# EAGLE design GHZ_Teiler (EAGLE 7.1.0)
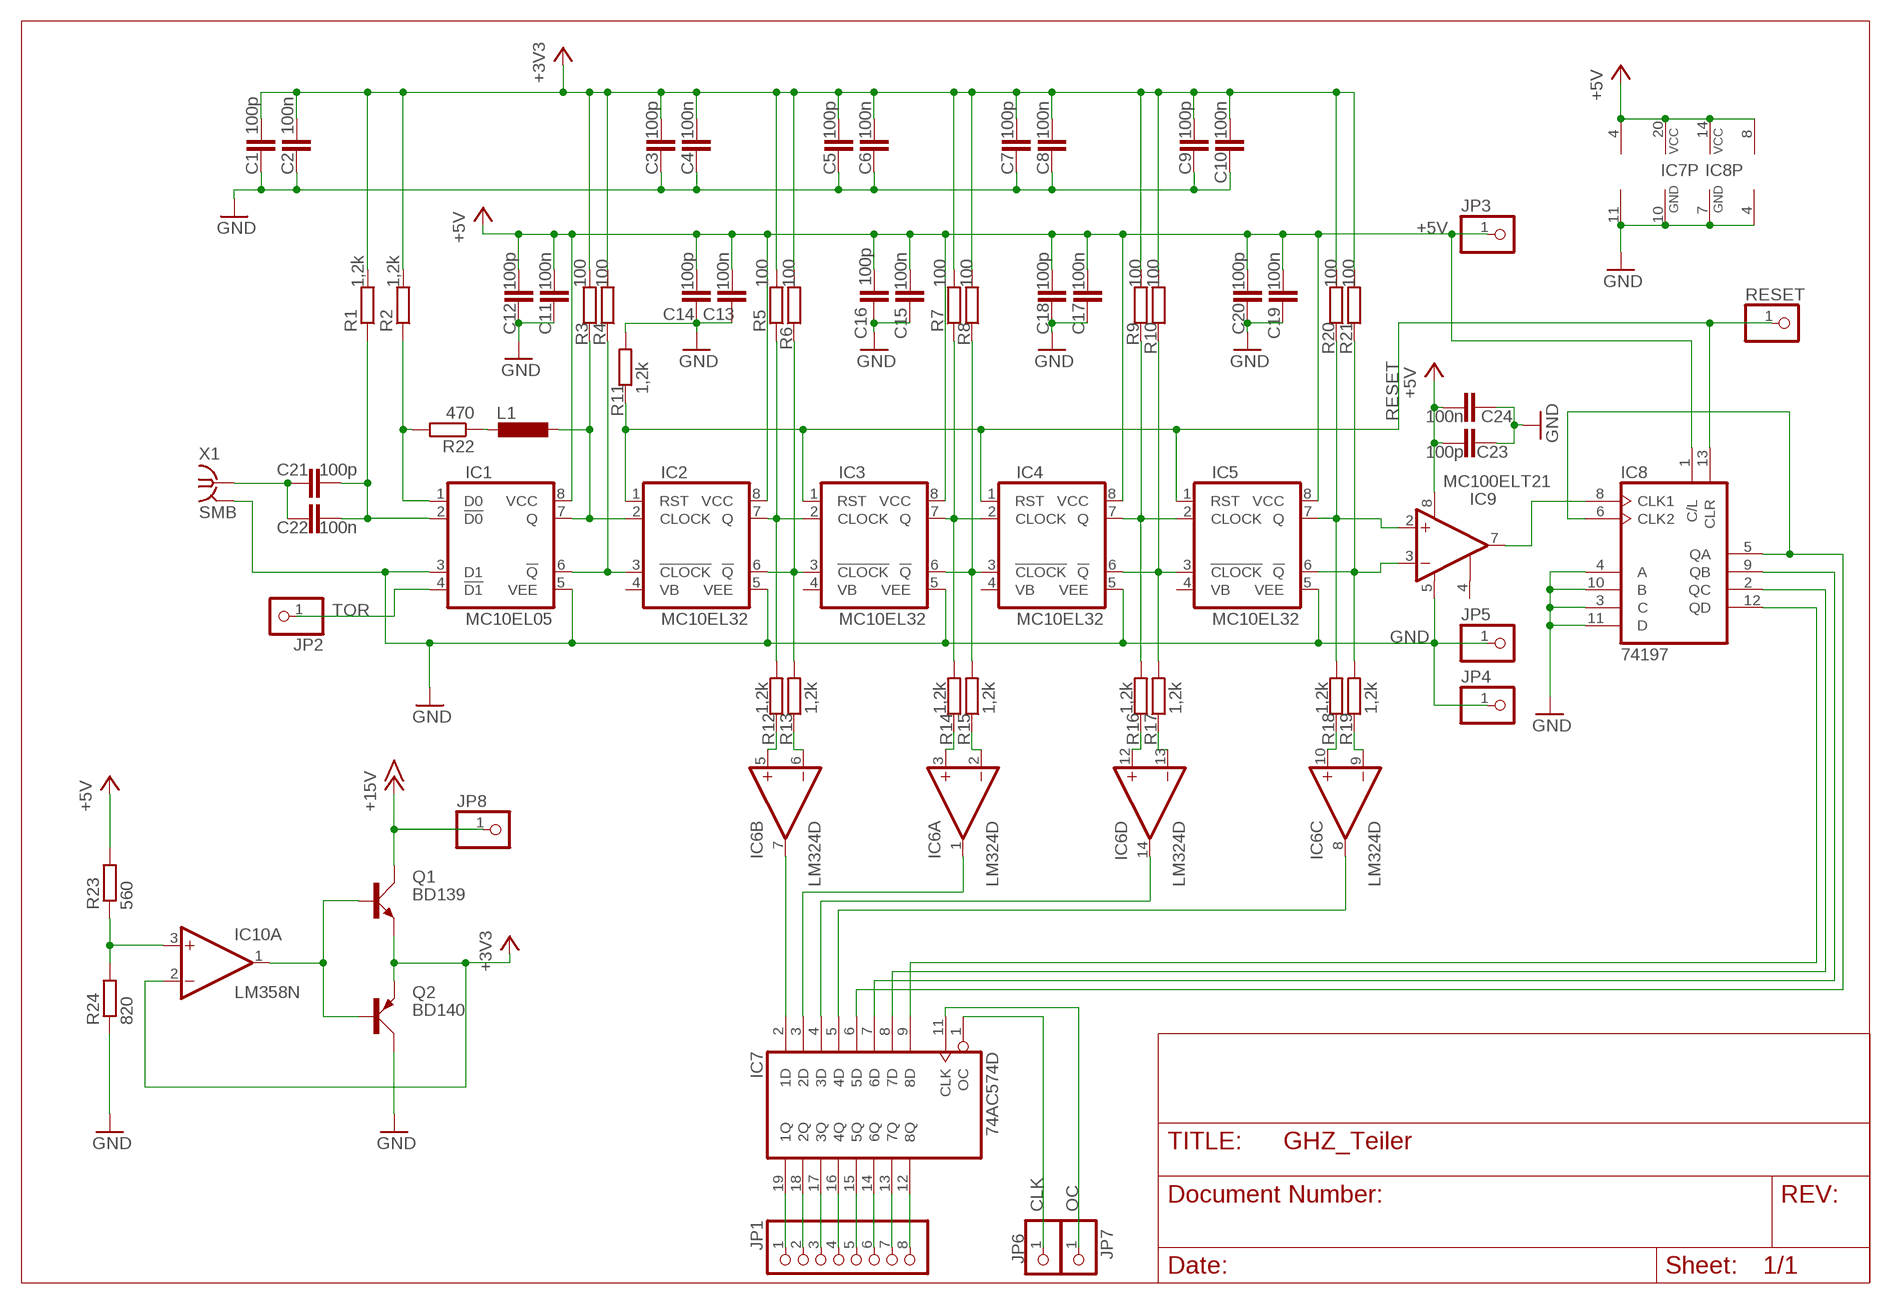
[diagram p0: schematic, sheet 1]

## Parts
C1  100p  C-EUC1206  [C1206]
C2  100n  C-EUC1206  [C1206]
C3  100p  C-EUC1206  [C1206]
C4  100n  C-EUC1206  [C1206]
C5  100p  C-EUC1206  [C1206]
C6  100n  C-EUC1206  [C1206]
C7  100p  C-EUC1206  [C1206]
C8  100n  C-EUC1206  [C1206]
C9  100p  C-EUC1206  [C1206]
C10  100n  C-EUC1206  [C1206]
C11  100n  C-EUC1206  [C1206]
C12  100p  C-EUC1206  [C1206]
C13  100n  C-EUC1206  [C1206]
C14  100p  C-EUC1206  [C1206]
C15  100n  C-EUC1206  [C1206]
C16  100p  C-EUC1206  [C1206]
C17  100n  C-EUC1206  [C1206]
C18  100p  C-EUC1206  [C1206]
C19  100n  C-EUC1206  [C1206]
C20  100p  C-EUC1206  [C1206]
C21  100p  C-EUC1206  [C1206]
C22  100n  C-EUC1206  [C1206]
C23  100p  C-EUC1206  [C1206]
C24  100n  C-EUC1206  [C1206]
IC1  MC10EL05  [SO8]
IC2  MC10EL32  [SO8]
IC3  MC10EL32  [SO8]
IC4  MC10EL32  [SO8]
IC5  MC10EL32  [SO8]
IC6  LM324D  [SO14]
IC7  74AC574D  [SO20W]
IC8  74197  74196  [DIL14]
IC9  MC100ELT21  [SO08]
IC10  LM358N  [DIL08]
JP1  PINHD-1X8  [1X08]
JP2  PINHD-1X1  [1X01]
JP3  PINHD-1X1  [1X01]
JP4  PINHD-1X1  [1X01]
JP5  PINHD-1X1  [1X01]
JP6  PINHD-1X1  [1X01]
JP7  PINHD-1X1  [1X01]
JP8  PINHD-1X1  [1X01]
L1  L-EUL2012C  [L2012C]
Q1  BD139  [TO126AV]
Q2  BD140  [TO126AV]
R1  1,2k  R-EU_M1206  [M1206]
R2  1,2k  R-EU_M1206  [M1206]
R3  100  R-EU_M1206  [M1206]
R4  100  R-EU_M1206  [M1206]
R5  100  R-EU_M1206  [M1206]
R6  100  R-EU_M1206  [M1206]
R7  100  R-EU_M1206  [M1206]
R8  100  R-EU_M1206  [M1206]
R9  100  R-EU_M1206  [M1206]
R10  100  R-EU_M1206  [M1206]
R11  1,2k  R-EU_M1206  [M1206]
R12  1,2k  R-EU_M1206  [M1206]
R13  1,2k  R-EU_M1206  [M1206]
R14  1,2k  R-EU_M1206  [M1206]
R15  1,2k  R-EU_M1206  [M1206]
R16  1,2k  R-EU_M1206  [M1206]
R17  1,2k  R-EU_M1206  [M1206]
R18  1,2k  R-EU_M1206  [M1206]
R19  1,2k  R-EU_M1206  [M1206]
R20  100  R-EU_M1206  [M1206]
R21  100  R-EU_M1206  [M1206]
R22  470  R-EU_M1206  [M1206]
R23  560  R-EU_M1206  [M1206]
R24  820  R-EU_M1206  [M1206]
RESET  PINHD-1X1  [1X01]
X1  SMB  BU-SMB-V  [BU-SMB-V]

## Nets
+3V3: C1.1 C2.1 C3.1 C4.1 C5.1 C6.1 C7.1 C8.1 C9.1 C10.1 IC10.2(A:-IN) Q1.E Q2.E R1.2 R2.2 R3.2 R4.2 R5.2 R6.2 R7.2 R8.2 R9.2 R10.2 R20.2 R21.2
+5V: C11.1 C12.1 C13.1 C14.1 C15.1 C16.1 C17.1 C18.1 C19.1 C20.1 C23.1 C24.1 IC1.8(VCC) IC2.8(VCC) IC3.8(VCC) IC4.8(VCC) IC5.8(VCC) IC6.4(P:V+) IC7.20(VCC) IC8.1(C/L) IC8.14(VCC) IC9.8(V+) IC10.8(P:V+) JP3.1 R23.2
+15V: JP8.1 Q1.C
CLK: IC7.1(OC) JP6.1
GND [Abstand]: C1.2 C2.2 C3.2 C4.2 C5.2 C6.2 C7.2 C8.2 C9.2 C10.2 C11.2 C12.2 C13.2 C14.2 C15.2 C16.2 C17.2 C18.2 C19.2 C20.2 C23.2 C24.2 IC1.3(D1) IC1.5(VEE) IC2.5(VEE) IC3.5(VEE) IC4.5(VEE) IC5.5(VEE) IC6.11(P:V-) IC7.10(GND) IC8.3(C) IC8.4(A) IC8.7(GND) IC8.10(B) IC8.11(D) IC9.5(V-) IC10.4(P:V-) JP4.1 JP5.1 Q2.C R11.2 R24.1 X1.2(GND)
N$1: IC1.1(D0) R2.1 R22.2
N$2: IC8.8(CLK1) IC9.7(OUT)
N$3: C21.2 C22.2 IC1.2(!D0) R1.1
N$4: C21.1 C22.1 X1.1
N$5: IC1.7(Q) IC2.2(CLOCK) L1.1 R3.1
N$6: IC1.6(!Q) IC2.3(!CLOCK) R4.1
N$7: IC2.7(Q) IC3.2(CLOCK) R5.1 R12.2
N$8: IC2.6(!Q) IC3.3(!CLOCK) R6.1 R13.2
N$9: IC3.7(Q) IC4.2(CLOCK) R7.1 R14.2
N$10: IC3.6(!Q) IC4.3(!CLOCK) R8.1 R15.2
N$11: IC4.7(Q) IC5.2(CLOCK) R9.1 R16.2
N$12: IC4.6(!Q) IC5.3(!CLOCK) R10.1 R17.2
N$13: IC6.5(B:+IN) R12.1
N$14: IC6.6(B:-IN) R13.1
N$15: IC6.3(A:+IN) R14.1
N$16: IC5.7(Q) IC9.2(+IN) R18.2 R20.1
N$17: IC5.6(!Q) IC9.3(-IN) R19.2 R21.1
N$18: IC6.2(A:-IN) R15.1
N$19: IC6.12(D:+IN) R16.1
N$20: IC6.13(D:-IN) R17.1
N$21: IC6.10(C:+IN) R18.1
N$22: IC6.9(C:-IN) R19.1
N$23: IC6.7(B:OUT) IC7.2(1D)
N$24: IC6.1(A:OUT) IC7.3(2D)
N$25: IC6.14(D:OUT) IC7.4(3D)
N$26: IC6.8(C:OUT) IC7.5(4D)
N$27: IC7.19(1Q) JP1.1
N$28: IC7.18(2Q) JP1.2
N$29: IC7.17(3Q) JP1.3
N$30: IC7.16(4Q) JP1.4
N$31: IC7.15(5Q) JP1.5
N$32: IC7.14(6Q) JP1.6
N$33: IC7.13(7Q) JP1.7
N$34: IC7.12(8Q) JP1.8
N$35: IC7.6(5D) IC8.5(QA) IC8.6(CLK2)
N$36: IC7.7(6D) IC8.9(QB)
N$37: IC7.8(7D) IC8.2(QC)
N$38: IC7.9(8D) IC8.12(QD)
N$39: IC10.3(A:+IN) R23.1 R24.2
N$40: L1.2 R22.1
N$41: IC10.1(A:OUT) Q1.B Q2.B
OC: IC7.11(CLK) JP7.1
RESET: IC2.1(RST) IC3.1(RST) IC4.1(RST) IC5.1(RST) IC8.13(CLR) R11.1 RESET.1
TOR: IC1.4(!D1) JP2.1
Unconnected: IC2.4(VB) IC3.4(VB) IC4.4(VB) IC5.4(VB) IC10.5(B:+IN) IC10.6(B:-IN) IC10.7(B:OUT)

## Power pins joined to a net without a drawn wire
GND: X1.3(GND) X1.4(GND) X1.5(GND)
VBB: IC9.4(VBB)

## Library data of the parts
C1-C24 = rcl:C-EU: CAPACITOR, European symbol
IC1 = 1Eigene:MC10EL05
IC2-IC5 = 1Eigene:MC10EL32
IC6 = linear:LM324: OP AMP
IC7 = 74xx-eu:74*574: 8-bit D type FLIP FLOP bus driver
IC8 = 1Eigene:74196
IC9 = 1Eigene:MC100ELT21
IC10 = linear:LM358: OP AMP also LM158; LM258; LM2904 Source: http://cache.national.com/ds/LM/LM158.pdf
JP1 = pinhead:PINHD-1X8: PIN HEADER
JP2-JP8 RESET = pinhead:PINHD-1X1: PIN HEADER
L1 = rcl:L-EU: INDUCTOR, European symbol
Q1 = transistor-power:BD139: NPN TRANSISTOR
Q2 = transistor-power:BD140: PNP TRANSISTOR
R1-R24 = rcl:R-EU_: RESISTOR, European symbol
X1 = con-coax:BU-SMB-V: FEMALE SMB CONNECTOR Radiall distributor RS 112-2993

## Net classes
1 Abstand: clearance 0.6 mm

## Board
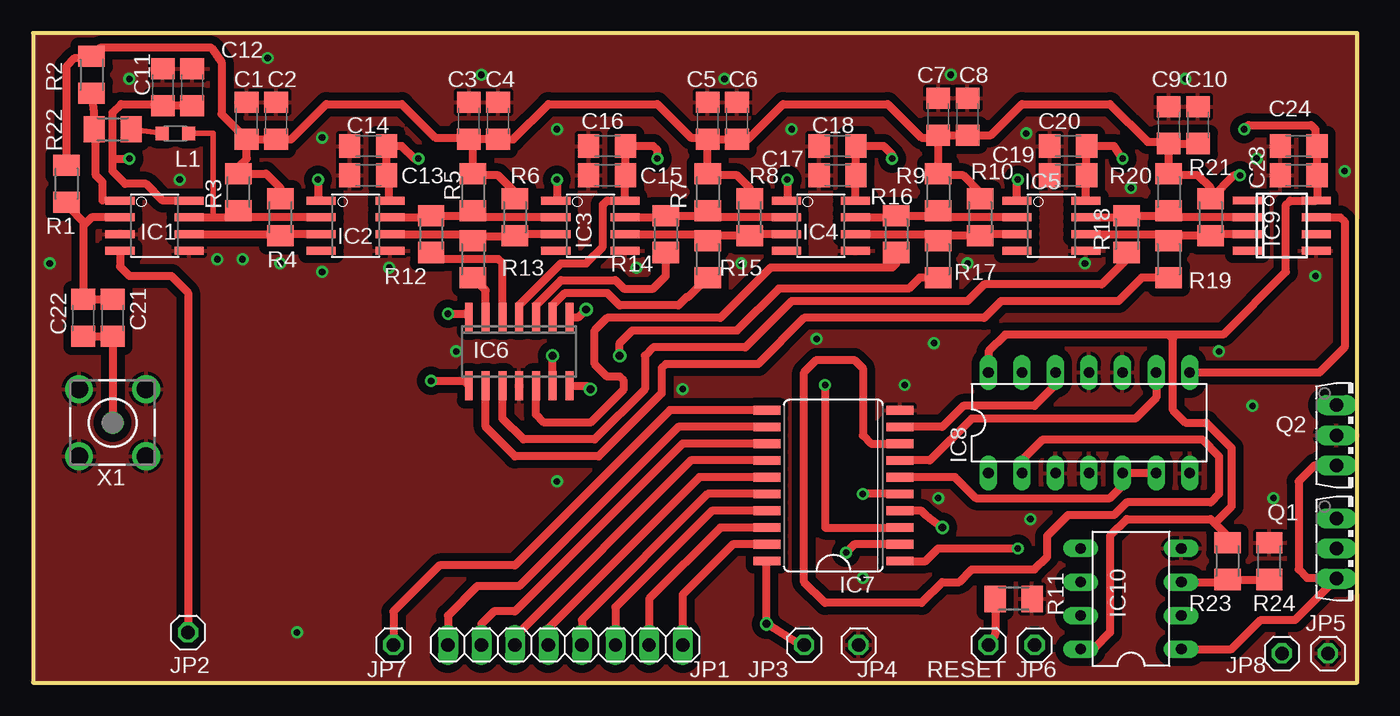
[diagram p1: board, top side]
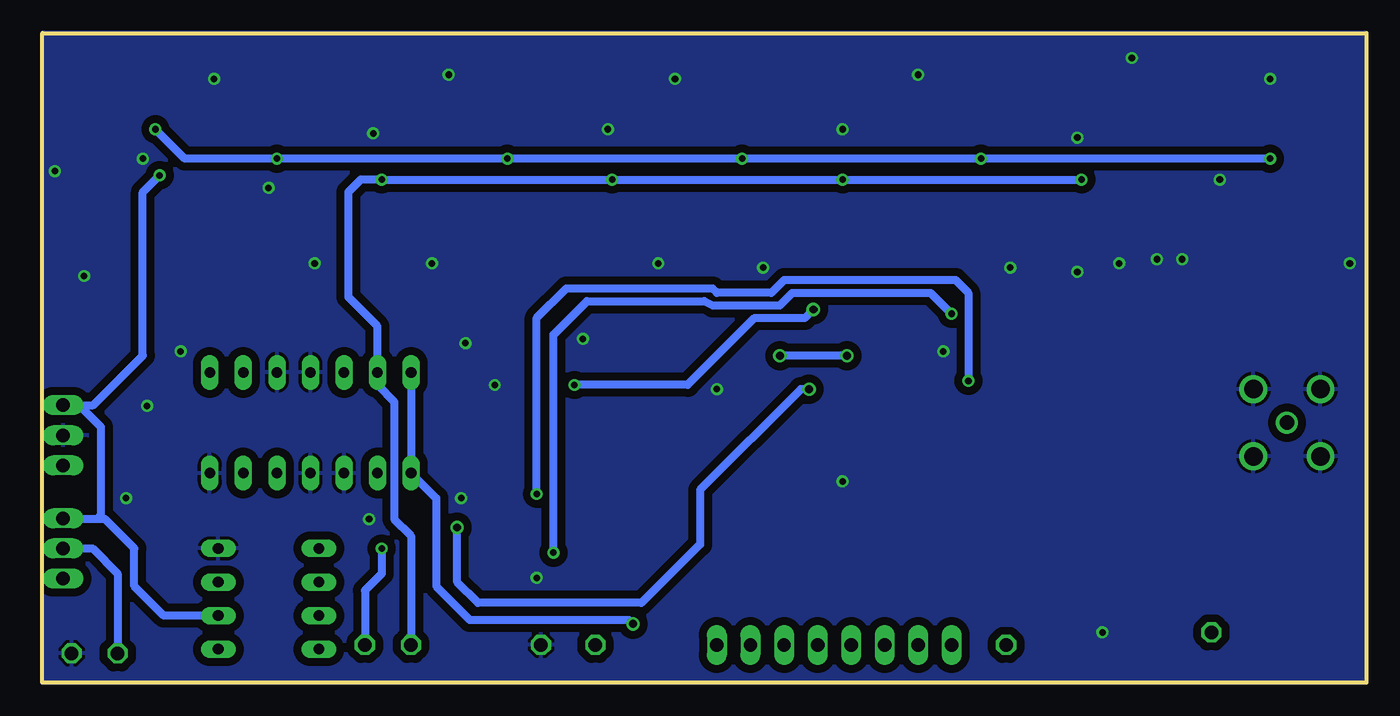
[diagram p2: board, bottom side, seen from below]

Size 100.31 x 49.2 mm. Coordinates in mm from the lower left corner, seen from the top.
Outline: 0,0 100.31,0 100.31,49.2 0,49.2 0,0
Copper layers (1*16): Top 0.035mm / dielectric 1.5mm / Bottom 0.035mm
Design rules "default *": minimum track width 0.6mm, minimum drill 0.5mm, track to track 0.2mm, track to pad 0.2mm, pad to pad 0.2mm, via to via 0.2mm, smd to smd 0.2mm, copper to edge 0mil, drill to drill 8mil, minimum pad ring 10mil, minimum via ring 8mil, stop-mask expansion 4mil, vias tented up to drill 0mil, thermal gap 10mil

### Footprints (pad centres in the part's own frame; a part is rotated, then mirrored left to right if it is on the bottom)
C1206 = smd 1.6 x 1.8: 1 -1.4,0; 2 1.4,0
SO8 = smd 0.61 x 2.21: 1 -1.905,-2.616; 2 -0.635,-2.616; 3 0.635,-2.616; 4 1.905,-2.616; 5 1.905,2.616; 6 0.635,2.616; 7 -0.635,2.616; 8 -1.905,2.616
SO14 = smd 0.6 x 2.2: 1 -3.81,-2.6; 2 -2.54,-2.6; 3 -1.27,-2.6; 4 0,-2.6; 5 1.27,-2.6; 6 2.54,-2.6; 7 3.81,-2.6; 8 3.81,2.6; 9 2.54,2.6; 10 1.27,2.6; 11 0,2.6; 12 -1.27,2.6; 13 -2.54,2.6; 14 -3.81,2.6
SO20W = smd 0.66 x 2.032: 1 -5.715,-5.029; 2 -4.445,-5.029; 3 -3.175,-5.029; 4 -1.905,-5.029; 5 -0.635,-5.029; 6 0.635,-5.029; 7 1.905,-5.029; 8 3.175,-5.029; 9 4.445,-5.029; 10 5.715,-5.029; 11 5.715,5.029; 12 4.445,5.029; 13 3.175,5.029; 14 1.905,5.029; 15 0.635,5.029; 16 -0.635,5.029; 17 -1.905,5.029; 18 -3.175,5.029; 19 -4.445,5.029; 20 -5.715,5.029
DIL14 = drill 0.813 long: 1 -6.35,-3.81; 2 -3.81,-3.81; 3 -1.27,-3.81; 4 1.27,-3.81; 5 3.81,-3.81; 6 6.35,-3.81; 7 8.89,-3.81; 8 8.89,3.81; 9 6.35,3.81; 10 3.81,3.81; 11 1.27,3.81; 12 -1.27,3.81; 13 -3.81,3.81; 14 -6.35,3.81
SO08 = smd 0.6 x 2.2: 1 -1.905,-2.6; 2 -0.635,-2.6; 3 0.635,-2.6; 4 1.905,-2.6; 5 1.905,2.6; 6 0.635,2.6; 7 -0.635,2.6; 8 -1.905,2.6
DIL08 = drill 0.813 long: 1 -3.81,-3.81; 2 -1.27,-3.81; 3 1.27,-3.81; 4 3.81,-3.81; 5 3.81,3.81; 6 1.27,3.81; 7 -1.27,3.81; 8 -3.81,3.81
1X08 = drill 1.016 long: 1 -8.89,0; 2 -6.35,0; 3 -3.81,0; 4 -1.27,0; 5 1.27,0; 6 3.81,0; 7 6.35,0; 8 8.89,0
1X01 = drill 1.016 octagon: 1 0,0
L2012C = smd 1 x 1: 1 -1,0; 2 1,0
TO126AV = drill 1.016 long: B 2.286,-1.27; C 0,-1.27; E -2.286,-1.27
M1206 = smd 1.6 x 2: 1 -1.4,0; 2 1.4,0
BU-SMB-V = drill 1.1: 1 0,0 | drill 1.4: 2 -2.54,2.54; 3 2.54,2.54; 4 2.54,-2.54; 5 -2.54,-2.54

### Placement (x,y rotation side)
C1  16.19,42.55 90 top
C2  18.41,42.55 90 top
C3  33.02,42.55 90 top
C4  35.24,42.55 90 top
C5  51.12,42.55 90 top
C6  53.34,42.55 90 top
C7  68.58,42.86 90 top
C8  70.8,42.86 90 top
C9  86.04,42.23 90 top
C10  88.27,42.23 90 top
C11  9.84,45.09 90 top
C12  12.06,45.09 90 top
C13  25.4,38.42 180 top
C14  25.4,40.64 180 top
C15  43.5,38.42 180 top
C16  43.5,40.64 180 top
C17  60.96,38.42 180 top
C18  60.96,40.64 180 top
C19  78.42,38.42 180 top
C20  78.42,40.64 180 top
C21  6.03,27.62 90 top
C22  3.81,27.62 90 top
C23  95.89,38.42 180 top
C24  95.89,40.64 180 top
IC1  9.21,34.61 270 top
IC2  24.45,34.61 270 top
IC3  42.23,34.61 270 top
IC4  59.69,34.61 270 top
IC5  77.15,34.61 270 top
IC6  36.83,25.08 180 top
IC7  60.64,14.92 90 top
IC8  78.74,19.68 0 top
IC9  94.61,34.61 270 top
IC10  83.19,6.35 90 top
JP1  40.32,2.86 180 top
JP2  11.75,3.81 90 top
JP3  58.42,2.86 90 top
JP4  62.55,2.86 90 top
JP5  98.11,2.22 90 top
JP6  75.88,2.86 90 top
JP7  27.3,2.86 90 top
JP8  94.61,2.22 90 top
L1  10.79,41.59 180 top
Q1  100.01,10.16 270 top
Q2  100.01,18.73 270 top
R1  2.54,37.78 90 top
R2  4.45,46.04 90 top
R3  15.56,37.15 90 top
R4  18.73,35.24 90 top
R5  33.34,37.15 90 top
R6  36.51,35.24 90 top
R7  51.12,37.15 90 top
R8  54.29,35.24 90 top
R9  68.58,37.15 90 top
R10  71.75,35.24 90 top
R11  74.3,6.35 0 top
R12  30.16,33.97 90 top
R13  33.34,32.07 90 top
R14  47.94,33.97 90 top
R15  51.12,32.07 90 top
R16  65.41,33.97 90 top
R17  68.58,32.07 90 top
R18  82.87,33.97 90 top
R19  86.04,32.07 90 top
R20  86.04,37.15 90 top
R21  89.22,35.24 90 top
R22  6.03,41.91 180 top
R23  90.49,9.21 90 top
R24  93.66,9.21 270 top
RESET  72.39,2.86 90 top
X1  6.03,19.68 90 top

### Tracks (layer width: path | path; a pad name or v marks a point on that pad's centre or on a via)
+3V3  (via drill 0.5)
  Top 0.6: R1.2 2.54,46.67 3.17,47.31 4.63,47.31 R2.2 5.08,48.07 13.52,48.07 14.29,46.99 14.29,43.05 C1.1 | C1.1 16.19,39.69 15.56,39.05 R3.2 17.65,38.55 18.73,37.47 R4.2 | C1.1 C2.1 19.55,41.15 22.23,43.81 27.94,43.81 30.48,41.27 32.89,41.27 C3.1 | C3.1 33.34,40.83 R5.2 33.47,38.42 35.24,38.42 36.51,37.15 | R6.2 36.51,37.15 | C3.1 C4.1 36.38,41.15 39.05,43.81 47.31,43.81 49.85,41.27 50.99,41.27 C5.1 | R8.2 54.29,37.47 53.34,38.42 51.25,38.42 R7.2 C5.1 | C5.1 C6.1 54.16,41.15 56.83,43.81 64.77,43.81 67.31,41.27 68.39,41.27 C7.1 | 36.51,37.15 36.2,37.15 | C7.1 R9.2 68.71,38.42 70.48,38.42 71.75,37.15 R10.2 | C7.1 C8.1 72.58,41.46 74.93,43.81 81.6,43.81 84.45,40.96 85.91,40.96 C9.1 | C9.1 R20.2 86.17,38.42 88.27,38.42 89.22,37.47 R21.2 90.99,38.42 v91.44,38.42 | C9.1 C10.1
  Bottom 0.6: v91.44,38.42 92.71,37.15 92.71,24.77 96.46,21.02 Q2.E 97.54,21.02 95.89,19.37 95.89,12.7 96.2,12.38 | IC10.2 91.12,5.08 93.34,7.3 93.34,10.16 95.57,12.38 96.2,12.38 | 96.2,12.38 98.68,12.38 Q1.E
+5V  (via drill 0.5, 0.6)
  Top 0.4: IC2.8 27.3,36.51
  Top 0.6: IC1.8 9.84,36.51 8.57,37.78 6.99,37.78 6.03,38.73 6.03,39.69 | 6.03,39.69 6.03,43.18 6.67,43.81 9.71,43.81 C11.1 C12.1 | IC2.8 26.99,36.59 26.99,38.23 C13.1 C14.1 | IC7.20 55.56,9.16 v55.56,4.45 58.1,2.86 JP3.1 | IC6.4 36.83,28.57 40.01,31.75 41.91,31.75 43.18,33.02 43.18,36.2 43.5,36.51 IC3.8 44.84,38.36 C15.1 C16.1 46.99,40.64 47.31,40.32 v47.31,39.69 | 26.67,40.77 C14.1 | IC4.8 62.31,38.36 C17.1 C18.1 64.45,40.64 65.09,40.01 v65.09,39.69 | IC5.8 79.77,38.36 C19.1 C20.1 81.92,40.64 v82.55,39.69 | 6.03,39.69 v7.3,39.69 | v29.21,39.69 28.89,39.69 27.94,40.64 C14.1 | v91.76,41.91 92.08,42.23 96.84,42.23 97.16,41.91 97.16,40.77 C24.1 C23.1 97.28,36.58 IC9.8 95.25,36.51 94.93,36.2 94.93,31.11 90.17,26.35 86.04,26.35 | 86.04,26.35 73.66,26.35 72.39,25.08 IC8.14 | 89.53,12.06 89.22,12.38 82.87,12.38 81.6,11.11 81.6,3.81 80.33,2.54 IC10.8 | 89.53,12.06 90.49,11.11 R23.2 | 86.04,26.35 86.36,26.04 86.36,20.64 87.31,19.68 88.9,19.68 90.81,17.78 90.81,13.34 89.53,12.06
  Bottom 0.6: IC8.14 IC8.1 70.48,13.97 70.48,7.3 67.94,4.76 55.88,4.76 v55.56,4.45 | v7.3,39.69 v29.21,39.69 v47.31,39.69 v65.09,39.69 v82.55,39.69 89.53,39.69 v91.76,41.91
+15V
  Bottom 0.6: Q1.C 96.52,10.16 94.61,8.26 JP8.1
CLK  (via drill 0.5)
  Top 0.6: IC7.1 67.63,9.21 68.58,10.16 v74.61,10.16
  Bottom 0.6: v74.61,10.16 74.61,8.26 75.88,6.99 JP6.1
GND  (via drill 0.5)
  Top 0.6: 94.8,38.4 C23.2
  other vias: 7.3,45.72 11.11,38.1 57.47,41.91 75.25,41.59 97.16,30.8 83.19,37.47 89.85,25.08 79.69,31.75 70.8,31.75 92.39,20.95 93.98,13.97 45.72,31.43 21.91,41.27 92.71,39.69 75.56,12.38 68.58,13.97 62.87,7.94 66.04,22.54 49.21,22.23 32.07,25.08 20,3.81 1.27,31.75 17.78,47.31 13.97,32.07 15.88,32.07 18.73,31.75 21.91,31.11 26.99,31.43 53.66,31.75 68.26,25.72 33.97,46.04 52.39,45.72 69.53,46.04 87.31,45.72 99.38,38.73 39.69,41.91 59.37,26.04 39.69,15.24
  pour Top: 0,0 0,49.21 100.33,49.21 100.33,0
  pour Bottom: 0,0 0,49.21 100.33,49.21 100.33,0
N$1
  Top 0.4: IC1.1 5.27,36.51
  Top 0.6: R2.1 4.63,43.24 R22.2 4.76,41.78 4.76,38.42 5.27,37.91 5.27,36.51
N$2
  Top 0.6: IC9.7 99.06,35.24 99.38,34.92 99.38,25.4 97.47,23.5 IC8.8
N$3
  Top 0.6: IC1.2 4.45,35.24 3.97,34.77 | 3.97,34.77 3.81,34.61 C22.2 C21.2 | R1.1 2.54,36.2 3.97,34.77
N$4
  Top 0.6: C22.1 C21.1 X1.1
N$5
  Top 0.4: 15.56,35.24 R3.1 | L1.1 13.65,41.59 13.65,35.24
  Top 0.6: IC1.7 13.65,35.24 15.56,35.24 IC2.2
N$6
  Top 0.4: 18.1,33.97 R4.1
  Top 0.6: IC1.6 18.1,33.97 | IC2.3 18.73,33.97 R4.1
N$7
  Top 0.4: 30.16,35.24 R12.2
  Top 0.6: IC2.7 30.16,35.24 | IC3.2 33.34,35.24 R5.1 33.34,35.37 R12.2
N$8
  Top 0.4: 33.34,33.97 R13.2 | 36.51,33.97 R6.1 36.51,33.78
  Top 0.6: IC2.6 33.34,33.97 | IC3.3 36.51,33.97 | 36.51,33.78 33.34,33.78 R13.2
N$9
  Top 0.6: IC3.7 47.94,35.24 R14.2 51.12,35.37 R7.1 51.12,35.24 IC4.2
N$10
  Top 0.6: IC3.6 51.12,33.97 51.12,33.84 | 51.12,33.84 R15.2 | 51.12,33.84 R8.1 54.29,33.97 IC4.3
N$11
  Top 0.6: IC4.7 65.41,35.24 R16.2 68.58,35.37 R9.1 68.58,35.24 IC5.2
N$12
  Top 0.6: IC4.6 68.58,33.97 68.58,33.84 | 68.58,33.84 R17.2 | 68.58,33.84 R10.1 71.75,33.97 IC5.3
N$13
  Top 0.6: IC6.5 35.56,31.75 35.24,32.07 30.67,32.07 R12.1
N$14
  Top 0.6: IC6.6 34.29,29.71 R13.1
N$15
  Top 0.6: IC6.3 38.1,28.57 40.01,30.48 44.13,30.48 44.77,29.84 46.99,29.84 47.94,30.8 R14.1
N$16
  Top 0.6: IC5.7 82.87,35.24 R18.2 86.04,35.37 R20.1 86.04,35.24 IC9.2
N$17
  Top 0.6: IC5.6 86.04,33.97 R19.2 | R19.2 86.36,33.47 86.36,33.34 | R19.2 86.04,33.84 R21.1 89.22,33.97 IC9.3
N$18
  Top 0.6: R15.1 49.66,29.21 49.53,29.21 48.9,28.57 44.45,28.57 43.5,29.53 40.32,29.53 39.37,28.57 IC6.2
N$19
  Top 0.6: R16.1 65.41,31.75 65.09,31.43 55.88,31.43 52.07,27.62 43.5,27.62 42.55,26.67 42.55,24.13 43.5,23.18 44.45,23.18 44.77,22.86 44.77,22.23 42.23,19.68 38.73,19.68 38.1,20.32 IC6.12
N$20  (via drill 0.6)
  Top 0.6: R17.1 67.18,30.67 66.36,29.84 56.52,29.84 53.34,26.67 45.4,26.67 44.45,25.72 v44.45,24.77 | IC6.13 v39.37,24.77
  Bottom 0.6: v39.37,24.77 v44.45,24.77
N$21
  Top 0.6: R18.1 82.87,32.07 80.96,30.16 72.07,30.16 70.8,28.89 57.47,28.89 53.98,25.4 46.99,25.4 46.35,24.77 46.35,22.23 42.55,18.41 37.15,18.41 35.56,20 IC6.10
N$22
  Top 0.6: R19.1 84.01,30.67 82.23,28.89 73.34,28.89 72.07,27.62 58.42,27.62 54.93,24.13 47.94,24.13 47.62,23.81 47.62,21.91 42.86,17.14 36.51,17.14 34.29,19.37 IC6.9
N$23  (via drill 0.5)
  Top 0.6: IC7.2 62.23,10.48 v61.59,9.84 | v31.43,27.94 32.76,27.94 IC6.7
  Bottom 0.6: v61.59,9.84 61.59,26.35 59.05,28.89 50.16,28.89 49.53,28.57 44.45,28.57 43.5,29.53 33.02,29.53 v31.43,27.94
N$24  (via drill 0.5, 0.6)
  Top 0.6: IC6.1 41.34,27.68 v41.91,28.26 | v60.01,22.54 60.01,11.75 IC7.3
  Bottom 0.6: v60.01,22.54 51.44,22.54 46.35,27.62 42.55,27.62 v41.91,28.26
N$25  (via drill 0.6)
  Top 0.6: IC6.14 41.97,22.48 v42.23,22.23 | v68.9,11.75 67.63,12.7 67.31,13.02 IC7.4
  Bottom 0.6: v42.23,22.23 42.86,22.23 50.48,14.61 50.48,10.48 54.93,6.03 67.31,6.03 68.9,7.62 v68.9,11.75
N$26  (via drill 0.5)
  Top 0.6: IC7.5 v62.87,14.29 | v30.16,22.86 32.64,22.86 IC6.8
  Bottom 0.6: v62.87,14.29 62.87,27.62 60.64,29.84 49.53,29.84 49.21,29.53 45.09,29.53 44.13,30.48 31.11,30.48 30.16,29.53 v30.16,22.86
N$27
  Top 0.6: IC7.19 53.02,10.48 49.21,6.67 JP1.1
N$28
  Top 0.6: IC7.18 52.07,11.75 46.67,6.35 JP1.2
N$29
  Top 0.6: IC7.17 51.44,13.02 44.13,5.71 JP1.3
N$30
  Top 0.6: IC7.16 51.12,14.29 41.59,4.76 JP1.4
N$31
  Top 0.6: IC7.15 50.48,15.56 39.05,4.13 JP1.5
N$32
  Top 0.6: IC7.14 49.85,16.83 36.51,3.49 JP1.6
N$33
  Top 0.6: IC7.13 49.21,18.1 36.51,5.4 34.92,5.4 33.97,4.45 JP1.7
N$34
  Top 0.6: IC7.12 48.9,19.37 36.83,7.3 33.66,7.3 31.43,5.08 JP1.8
N$35
  Top 0.6: IC8.6 IC8.5 82.55,14.92 81.6,13.97 71.44,13.97 69.85,15.56 IC7.6
N$36
  Top 0.6: IC8.9 85.09,21.59 83.5,20 71.12,20 67.94,16.83 IC7.7
N$37
  Top 0.6: IC8.2 74.93,16.83 76.52,18.41 88.58,18.41 89.85,17.14 89.85,14.29 89.22,13.65 82.87,13.65 81.92,12.7 78.42,12.7 76.83,11.11 76.83,9.53 75.88,8.57 71.12,8.57 70.17,7.62 68.9,7.62 67.31,6.03 60.01,6.03 58.42,7.62 58.42,23.5 59.37,24.45 62.23,24.45 62.87,23.81 62.87,18.73 63.5,18.1 IC7.8
N$38
  Top 0.6: IC8.12 77.47,22.54 75.88,20.95 70.48,20.95 68.9,19.37 IC7.9
N$39
  Top 0.6: IC10.3 90.3,7.62 R23.1 R24.2
N$40
  Top 0.4: L1.2 R22.1
N$41
  Top 0.6: Q2.B 97.09,16.45 95.89,15.24 95.89,8.57 96.52,7.94 98.68,7.94 Q1.B 95.63,4.76 93.03,4.76 90.81,2.54 IC10.1
OC
  Top 0.6: IC7.11 48.26,20.64 36.51,8.89 30.8,8.89 27.3,5.4 JP7.1
RESET  (via drill 0.5)
  Top 0.6: IC5.1 74.54,38.02 v74.61,38.1 | v57.15,38.1 57.15,36.59 IC4.1 | v39.69,38.1 39.69,36.59 IC3.1 | v21.59,38.1 21.59,36.75 IC2.1 | R11.1 72.89,3.68 RESET.1
  Bottom 0.6: v21.59,38.1 v39.69,38.1 v57.15,38.1 v74.61,38.1 76.2,38.1 77.15,37.15 77.15,29.21 74.93,26.99 IC8.13 74.93,22.54 73.66,21.27 73.66,12.38 72.39,11.11 RESET.1
TOR
  Top 0.6: IC1.4 6.59,31.51 7.3,30.8 10.48,30.8 11.75,29.53 JP2.1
